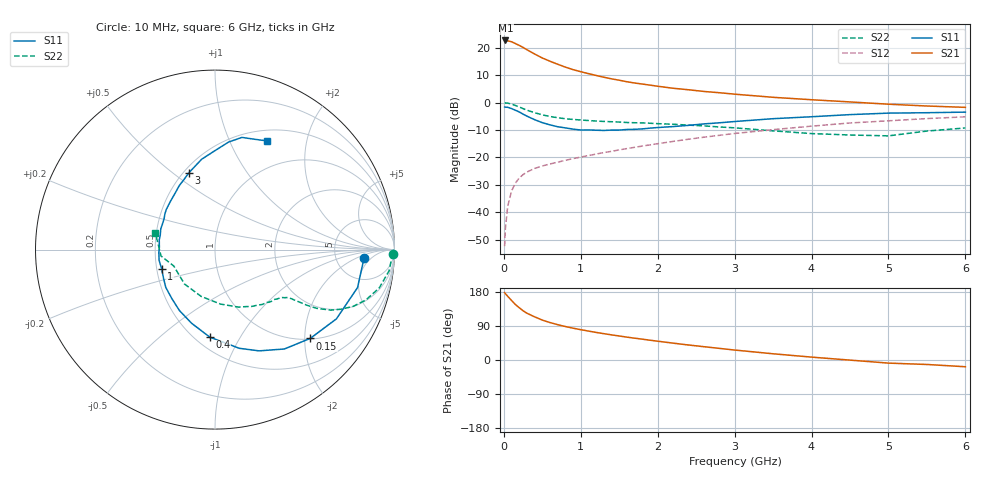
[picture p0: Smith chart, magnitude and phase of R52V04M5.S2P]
! SIEMENS Small Signal Semiconductors
! BFR183
! Si NPN RF Bipolar Junction Transistor in SOT23
! VCE = 2 V  IC = 4.5 mA
! Common Emitter S-Parameters:  May  1996
# GHz  S  MA  R  50
!  f  S11  S21  S12  S22
! GHz  MAG  ANG  MAG  ANG  MAG  ANG  MAG  ANG
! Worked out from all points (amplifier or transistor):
!   36 points, 10 MHz to 6 GHz, reference 50 ohm
!   highest |S21| = 22.7 dB at 20 MHz (marker M1)
!   |S21| within 3 dB of that: start of sweep to 277.4 MHz
!   unconditionally stable (mu >= 1): 1.079 GHz to 2.669 GHz
!   at 250 MHz: K = 0.40, MSG = 23.2 dB, |S12| = -26.3 dB
!   at 1.4 GHz: K = 1.06, MAG = 11.7 dB, |S12| = -17.8 dB
!   at 6 GHz: K = 0.89, MSG = 1.7 dB, |S12| = -5.2 dB
!   S11 on the Smith chart (normalised r, x): 10 MHz: 10, -3; 150 MHz: 1.02, -2.13; 400 MHz: 0.59, -0.75; 1 GHz: 0.53, -0.13; 3 GHz: 0.53, +0.57; 6 GHz: 0.63, +1.39
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0.01  0.8319 -3.2  13.61 177.8  0.0024 89.0  0.9922 -1.3
0.02  0.8263 -6.0  13.62 175.1  0.005 84.2  0.9854 -2.8
0.05  0.822 -14.9  13.41 168.2  0.0127 82.3  0.9775 -6.9
0.1  0.7788 -29.7  12.91 157.1  0.0243 74.7  0.9399 -13.1
0.15  0.7256 -43.0  11.96 146.5  0.0339 68.5  0.8869 -18.4
0.2  0.6752 -55.1  11.08 137.9  0.0421 64.5  0.8329 -22.3
0.25  0.6152 -66.5  10.16 129.9  0.0486 60.3  0.7773 -25.3
0.3  0.5662 -76.2  9.236 123.5  0.0541 58.2  0.7276 -27.6
0.4  0.4885 -93.4  7.709 113.9  0.0629 54.7  0.6547 -30.0
0.5  0.4304 -107.7  6.519 105.3  0.0697 53.7  0.5983 -31.2
0.6  0.3928 -120.4  5.686 98.8  0.0758 53.3  0.5581 -31.8
0.7  0.3627 -131.8  5.012 93.2  0.0818 53.6  0.5298 -32.3
0.8  0.3459 -142.4  4.443 88.3  0.0885 54.1  0.5075 -32.7
1  0.316 -160.3  3.662 80.0  0.1013 55.0  0.4817 -33.7
1.1  0.3172 -169.0  3.38 76.3  0.1082 55.9  0.4708 -34.7
1.6  0.3235 159.0  2.404 60.3  0.1451 57.2  0.4336 -39.7
2.2  0.3655 133.0  1.828 44.5  0.1958 55.9  0.4034 -49.2
3  0.4517 108.9  1.426 26.3  0.2734 50.0  0.3464 -67.7
3.5  0.5089 98.4  1.25 16.4  0.321 44.7  0.305 -84.2
4.5  0.6039 82.8  1.029 -0.3  0.425 32.6  0.2563 -131.5
5.5  0.654 69.9  0.867 -11.8  0.5112 19.9  0.3028 -173.3
6  0.6707 64.6  0.819 -17.8  0.5502 11.5  0.3448 164.4
